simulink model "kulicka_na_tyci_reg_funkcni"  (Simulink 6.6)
settings: Solver=FixedStepDiscrete  StartTime=0.0  StopTime=inf  FixedStep=0.01  RelTol=1e-3
undefined symbols (not defined in the file or in its folder): Humusoft, MF624, to, V
libraries: rtlib x4, simulink x1

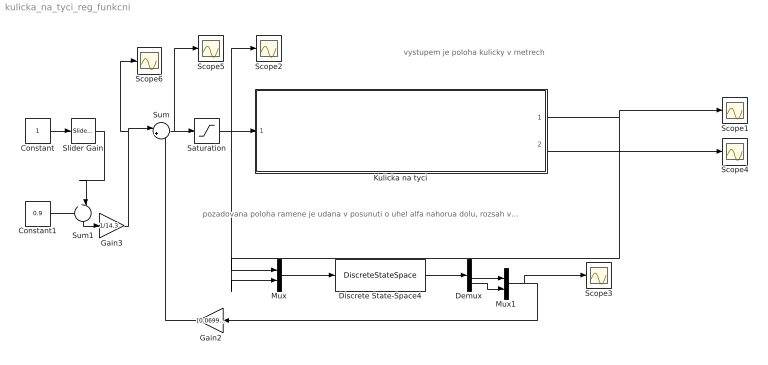
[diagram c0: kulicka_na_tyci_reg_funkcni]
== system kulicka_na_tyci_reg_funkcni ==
  note: pozadovana poloha ramene je udana v posunuti o uhel alfa nahorua dolu, rozsah vstupu do soustavy je: [-0.01 ; 0.01] , kde 0 je nulova odchylka ramene
  note: vystupem je poloha kulicky v metrech
  Constant : Constant
  Constant1 : Constant  Value=0.9
  Demux : Demux  Outputs=3
  Discrete State-Space4 : DiscreteStateSpace  A="[0.92516705771090   0.02000000000000;-0.13499379805524   1.00000000000000]"  B="[0.00140142857143   0.07483294228910;0.14014285714286   0.13499379805524]"  C="[0.92786693367201 0;0.92786693367201 0;-0.13499379805524  1.00000000000000]"  D="[0 0.07213306632799; 0   0.07213306632799;0   0.13499379805524]"  SampleTime=0.01
  Gain2 : Gain  Orientation=left  Gain="[0.06992876198436   0.15763664365243]"  Multiplication=Matrix(K*u)
  Gain3 : Gain  Gain=1/14.3
  Kulicka na tyci : Subsystem  TreatAsAtomicUnit=on  mask{Ts=0.01, IN_K=1, IN_R=2, OUT_S=1}
      mask prompts: Ts "Vzorkovaci perioda [s]"; IN_K "Cislo analog. vstupu - poloha kulicky"; IN_R "Cislo analog. vstupu - poloha ramane"; OUT_S "Cislo analog vystutpu - rizeni naklonu"
  Mux : Mux  Inputs=2
  Mux1 : Mux  Inputs=2
  Saturation : Saturate  UpperLimit=0.01  LowerLimit=-0.01  SampleTime=0.01
  Scope{1..6} (6 alike) : Scope
  Slider Gain : simulink/Math Operations/Slider Gain  SystemSampleTime=-1  low=0.1  gain=0.5  high=1
  Sum : Sum  Inputs=|+-
  Sum1 : Sum  Orientation=down  Inputs=+-|
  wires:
  Kulicka na tyci/1(kulicka) -> Scope1/1, Mux/2
  Constant/1 -> Slider Gain/1
  Mux/1 -> Discrete State-Space4/1
  Discrete State-Space4/1 -> Demux/1
  Demux/3 -> Mux1/2
  Demux/2 -> Mux1/1
  Mux1/1 -> Gain2/1, Scope3/1
  Gain2/1 -> Sum/2
  Sum/1 -> Saturation/1, Scope5/1
  Saturation/1 -> Kulicka na tyci/1(rameno), Mux/1, Scope2/1
  Constant1/1 -> Sum1/1
  Sum1/1 -> Gain3/1
  Kulicka na tyci/2(rameno out) -> Scope4/1
  Slider Gain/1 -> Sum1/2
  Gain3/1 -> Sum/1, Scope6/1

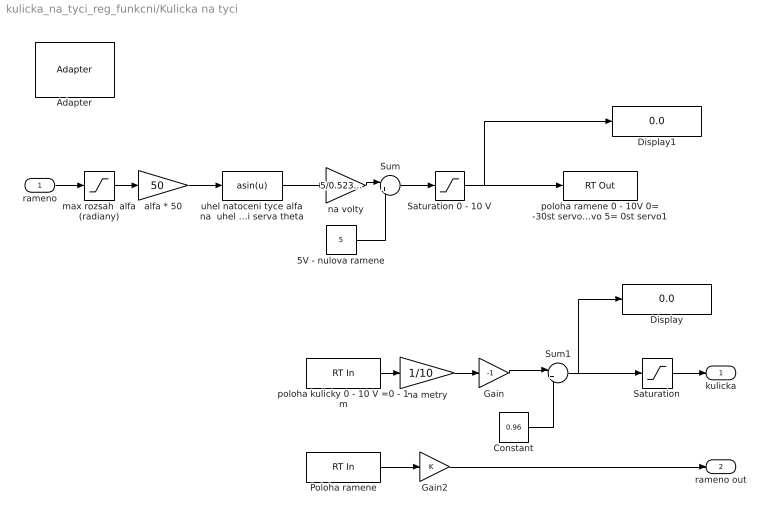
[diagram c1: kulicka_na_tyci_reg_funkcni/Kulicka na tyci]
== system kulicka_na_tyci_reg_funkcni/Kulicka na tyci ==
  rameno : Inport
  5V - nulova ramene : Constant  Value=5
  Adapter : rtlib/Adapter  SystemSampleTime=-1  DriverName=Humusoft/MF624  DriverAddress=4294967295  DriverOptions=0
  Constant : Constant  Value=0.96
  Display : Display
  Display1 : Display
  Gain : Gain  Gain=-1
  Gain2 : Gain
  Poloha ramene : rtlib/RT In  SampleTime=Ts  Adapter=Adapter  IOClass=Analog Input  Channels=IN_R  SLDataType=double  MaxMissedTicks=100  ShowMissedTicks=off  YieldWhenWaiting=on  AIORange=-10 to 10 V  AIOUnits=Volts  DIOMode=Bit  CIReset=never  CIEdge=rising  CIGate=none  EIQuadrature=quadruple  EIIndexPulse=reset  EIFilterFrequency=Inf  OIOParameters=[]
  Saturation : Saturate  UpperLimit=0.95  LowerLimit=0
  Saturation 0 - 10 V : Saturate  UpperLimit=10  LowerLimit=0
  Sum : Sum  Inputs=|++
  Sum1 : Sum  Inputs=|++
  alfa * 50 : Gain  Gain=50
  max rozsah  alfa (radiany) : Saturate  UpperLimit=0.01  LowerLimit=-0.01
  na metry : Gain  Gain=1/10
  na volty : Gain  Gain=5/0.52359877559830
  poloha kulicky 0 - 10 V =0 - 1 m : rtlib/RT In  SampleTime=Ts  Adapter=Adapter  IOClass=Analog Input  Channels=IN_K  SLDataType=double  MaxMissedTicks=100  ShowMissedTicks=off  YieldWhenWaiting=on  AIORange=-10 to 10 V  AIOUnits=Volts  DIOMode=Bit  CIReset=never  CIEdge=rising  CIGate=none  EIQuadrature=quadruple  EIIndexPulse=reset  EIFilterFrequency=Inf  OIOParameters=[]
  poloha ramene 0 - 10V 0= -30st servo 10= +30st servo 5= 0st servo1 : rtlib/RT Out  SampleTime=Ts  Adapter=Adapter  IOClass=Analog Output  Channels=OUT_S  InitialValue=[0]  FinalValue=[0]  MaxMissedTicks=100  ShowMissedTicks=off  YieldWhenWaiting=on  AIORange=-10 to 10 V  AIOUnits=Volts  DIOMode=Bit  OIOParameters=[]
  uhel natoceni tyce alfa na  uhel natoceni serva theta : Fcn  Expr=asin(u)
  kulicka : Outport
  rameno out : Outport  Port=2
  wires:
  poloha kulicky 0 - 10 V =0 - 1 m/1 -> na metry/1
  rameno/1 -> max rozsah  alfa (radiany)/1
  Saturation 0 - 10 V/1 -> Display1/1, poloha ramene 0 - 10V 0= -30st servo 10= +30st servo 5= 0st servo1/1
  Poloha ramene/1 -> Gain2/1
  Gain2/1 -> rameno out/1
  uhel natoceni tyce alfa na  uhel natoceni serva theta/1 -> na volty/1
  alfa * 50/1 -> uhel natoceni tyce alfa na  uhel natoceni serva theta/1
  max rozsah  alfa (radiany)/1 -> alfa * 50/1
  na volty/1 -> Sum/1
  5V - nulova ramene/1 -> Sum/2
  Sum/1 -> Saturation 0 - 10 V/1
  na metry/1 -> Gain/1
  Saturation/1 -> kulicka/1
  Gain/1 -> Sum1/1
  Sum1/1 -> Saturation/1, Display/1
  Constant/1 -> Sum1/2
